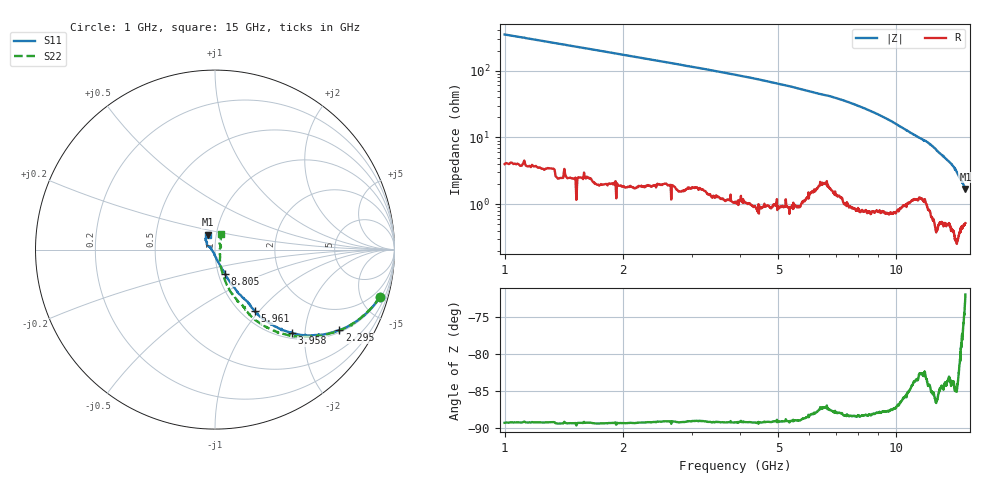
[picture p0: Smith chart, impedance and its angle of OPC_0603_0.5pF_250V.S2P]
! FILE NAME
! DATE 08/22/2012  10:02
! CORRECTED  DATA
# GHz  S  MA  R  50.00
!  FREQ  S11M  S11A  S21M  S21A  S12M  S12A  S22M  S22A
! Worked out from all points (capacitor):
!   1601 points, 1 GHz to 15 GHz, reference 50 ohm
!   read as one part in series: C = 458 fF near 1.07 GHz
!   lowest |Z| = 1.7 ohm at 15 GHz (marker M1)
!   S11 on the Smith chart (normalised r, x): 1 GHz: 1.13, -6.91; 2.295 GHz: 1.08, -3.03; 3.958 GHz: 1.10, -1.72; 5.961 GHz: 1.16, -0.95; 8.805 GHz: 1.08, -0.29; 15 GHz: 0.91, +0.15
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1  0.9559 -16.1  0.2747 73.4  0.2747 73.4  0.9558 -16.0
1.5775  0.9037 -24.2  0.4105 65.2  0.4106 65.1  0.9038 -24.2
2.295  0.8255 -33.0  0.5492 56.3  0.5493 56.4  0.8253 -33.2
3.33625  0.7065 -42.6  0.6947 46.2  0.6947 46.3  0.705 -43.5
3.9575  0.6341 -47.3  0.7618 41.3  0.7618 41.3  0.6331 -48.8
5.6725  0.4411 -56.4  0.8861 30.6  0.8863 30.7  0.4401 -60.8
5.96125  0.4075 -56.9  0.8975 29.0  0.8963 29.1  0.4081 -61.8
8  0.2162 -64.1  0.9655 21.0  0.9648 21.1  0.2165 -71.3
8.805  0.145 -67.3  0.9793 18.2  0.9788 18.3  0.148 -72.3
9.715  0.07891 -74.2  0.9865 15.5  0.9865 15.5  0.08156 -68.5
10.33625  0.04102 -85.1  0.987 13.7  0.9868 13.8  0.04863 -53.9
10.84375  0.02003 -110.1  0.9838 12.5  0.9837 12.6  0.03034 -31.2
11.10625  0.01592 -142.4  0.9806 12.1  0.9806 12.2  0.0249 -5.2
11.47375  0.01914 171.8  0.9823 11.5  0.9819 11.6  0.03272 19.3
11.61375  0.0228 165.3  0.9823 11.3  0.9825 11.4  0.03542 24.3
11.745  0.02841 160.1  0.982 11.1  0.9835 10.7  0.03685 24.6
11.9725  0.02872 153.8  0.9862 10.8  0.9858 10.8  0.0364 35.0
12.6725  0.05603 145.1  0.9855 9.5  0.9858 9.6  0.04753 59.3
13.0925  0.06141 138.0  0.9873 8.9  0.9872 8.9  0.05968 60.2
14.195  0.08201 128.0  0.9919 7.5  0.9919 7.6  0.07714 63.1
14.44  0.07969 123.2  0.9923 6.9  0.9924 7.0  0.07763 65.9
15  0.09314 116.6  0.9914 6.8  0.9916 6.9  0.09547 69.2
